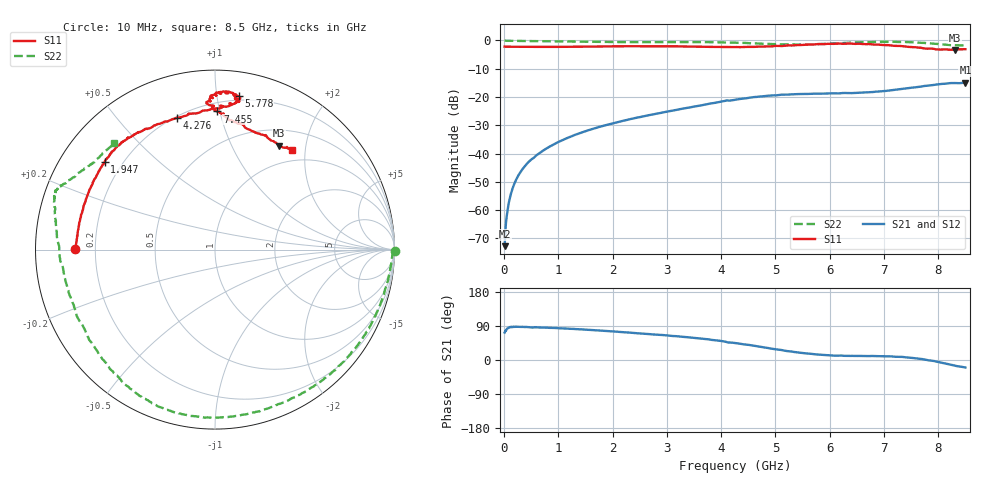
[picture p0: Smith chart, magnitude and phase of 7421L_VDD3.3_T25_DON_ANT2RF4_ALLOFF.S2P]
!Agilent Technologies,E5071C,MY46417908,A.11.23
!Date: Thu Feb 25 16:17:42 2021
!Data & Calibration Information:
!Freq	S11:SOLT2(ON)	S21:SOLT2(ON)	S12:SOLT2(ON)	S22:SOLT2(ON)
!PortZ  Port1:50+j0  Port2:50+j0
!Above PortZ is port z conversion or system Z0 setting when saving the data.
!When reading, reference impedance value at option line is always used.
# Hz S dB R 50
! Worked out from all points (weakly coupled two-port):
!   1601 points, 10 MHz to 8.5 GHz, reference 50 ohm
!   highest |S21| = -14.93 dB at 8.5 GHz (marker M1); lowest = -72.8 dB at 10 MHz (marker M2)
!   lowest |S11| = -3.3 dB at 8.309 GHz (marker M3), VSWR 5.26, Z = 36 + j77.5 ohm
!   |S11| at or under -10 dB: nowhere
!   |S22| runs from -1.8 to 0.0 dB; largest |S21 - S12| = 0.0029
!   S11 on the Smith chart (normalised r, x): 10 MHz: 0.12, +0.00; 1.947 GHz: 0.13, +0.34; 4.276 GHz: 0.21, +0.73; 5.778 GHz: 0.17, +1.15; 7.455 GHz: 0.26, +0.98; 8.5 GHz: 0.81, +1.75
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1e7  -2.18 179.7  -72.79 72.3  -71.80 75.8  0.00 -0.4
7.3675e7  -2.22 178.5  -59.01 84.4  -58.85 83.4  -0.11 -2.2
1.267375e8  -2.22 177.5  -54.20 86.6  -54.30 87.0  -0.13 -3.6
2.169438e8  -2.25 175.5  -49.47 88.1  -49.46 88.0  -0.15 -5.9
3.442938e8  -2.26 173.0  -45.45 87.3  -45.40 87.3  -0.18 -9.2
4.7695e8  -2.27 170.3  -42.52 86.1  -42.52 86.1  -0.23 -12.7
7.634875e8  -2.28 164.6  -38.42 85.3  -38.42 85.4  -0.29 -20.0
1.426769e9  -2.19 151.0  -32.61 80.8  -32.60 80.8  -0.43 -38.0
1.946781e9  -2.10 141.4  -29.60 75.9  -29.59 75.8  -0.53 -53.1
2.843538e9  -2.02 131.1  -25.81 66.6  -25.82 66.6  -0.60 -80.3
3.512125e9  -2.15 123.2  -23.34 58.3  -23.33 58.2  -0.57 -99.1
4.255e9  -2.35 106.9  -20.98 44.9  -20.98 44.9  -0.78 -118.4
4.276225e9  -2.33 106.3  -20.91 44.4  -20.91 44.4  -0.80 -119.0
4.960731e9  -2.02 87.3  -19.41 29.0  -19.38 28.9  -1.28 -141.7
5.671769e9  -1.46 81.8  -18.84 16.1  -18.78 16.4  -1.39 -172.1
5.777894e9  -1.27 81.2  -18.83 14.4  -18.83 14.7  -1.27 -175.8
6.41995e9  -1.17 88.4  -18.60 10.8  -18.65 11.2  -0.74 166.4
7.088538e9  -1.63 92.3  -17.72 10.0  -17.79 9.7  -0.47 160.2
7.454669e9  -2.27 89.0  -16.90 6.4  -16.89 6.5  -0.63 157.8
7.704062e9  -2.67 84.8  -16.26 2.5  -16.26 2.5  -0.85 155.2
8.308975e9  -3.34 58.2  -15.07 -15.0  -15.07 -15.3  -1.67 140.7
8.5e9  -3.10 52.1  -14.93 -19.9  -15.02 -20.3  -1.78 133.5
